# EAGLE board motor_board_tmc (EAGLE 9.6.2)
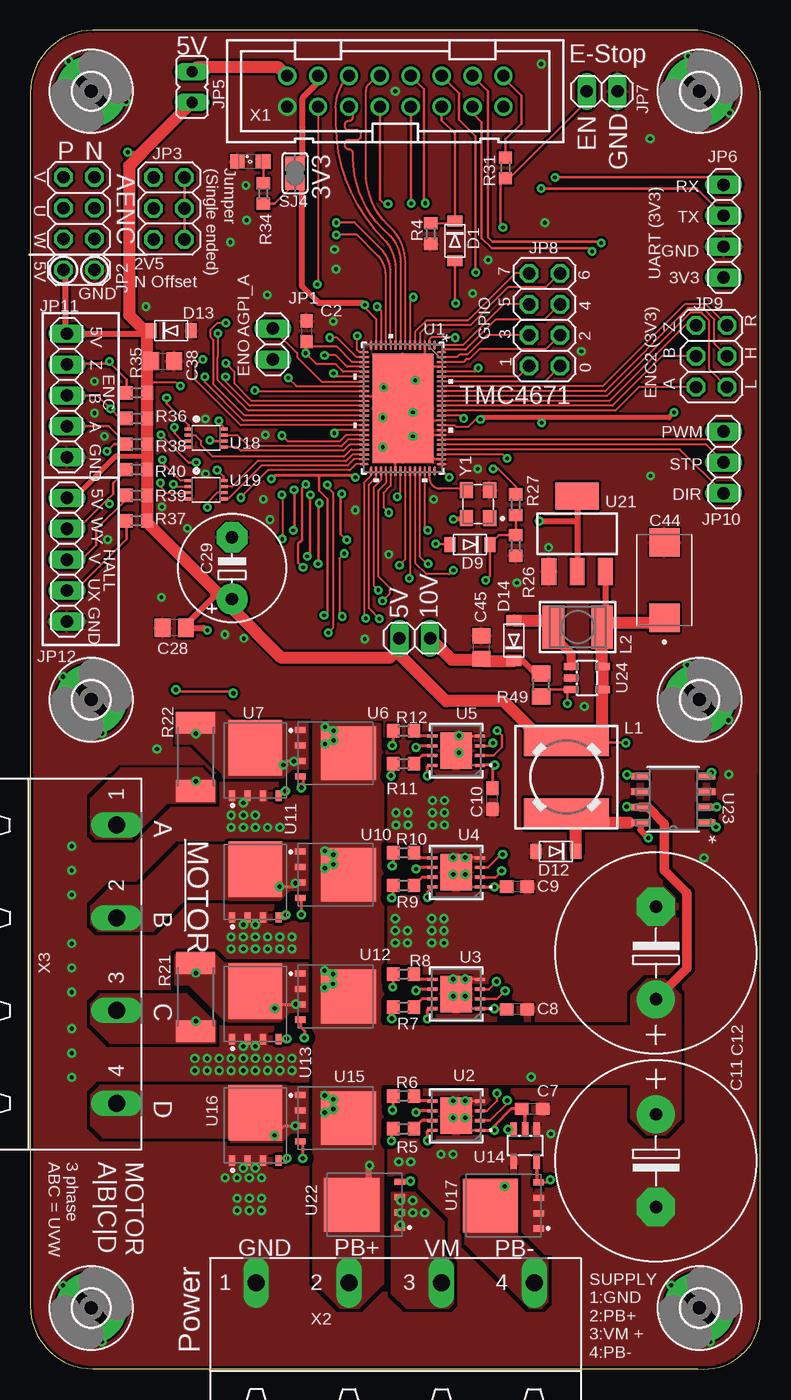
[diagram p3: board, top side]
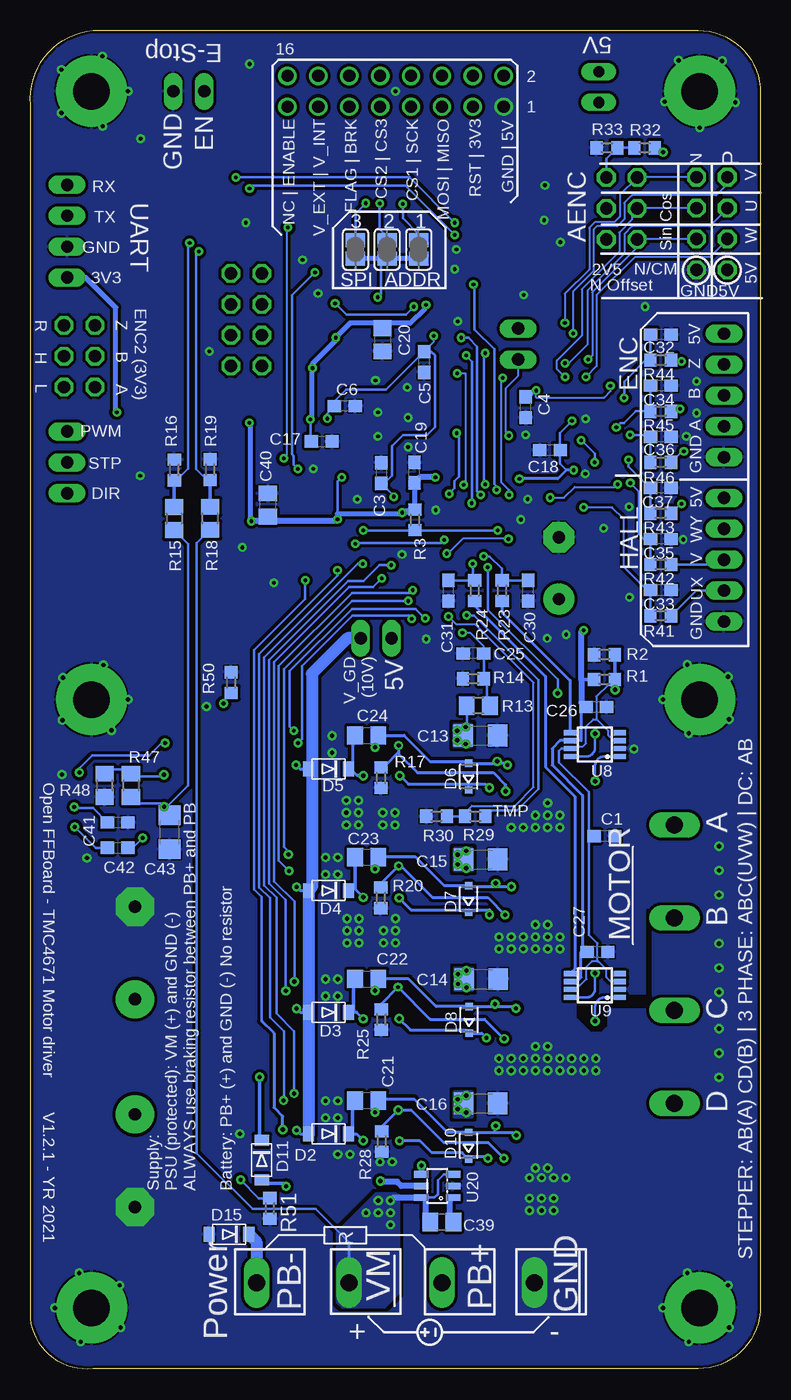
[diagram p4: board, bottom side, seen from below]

Size 60.02 x 110.03 mm. Coordinates in mm from the lower left corner, seen from the top.
Outline: 0,104.91 0,5.15 arc90 5.12,0.03 54.88,0.03 arc90 60,4.15 60,103.91 arc90 54.88,110.03 5.12,110.03 arc90 0,104.91
Copper layers (1*16): Top 0.035mm / dielectric 1.5mm / Bottom 0.035mm
Design rules "jlcpcb *": minimum track width 5mil, minimum drill 0.3mm, track to track 8mil, track to pad 8mil, pad to pad 8mil, via to via 8mil, smd to smd 5mil, copper to edge 0.2mm, drill to drill 8mil, minimum pad ring 10mil, minimum via ring 8mil, stop-mask expansion 4mil, vias tented up to drill 0.4mm, thermal gap 6mil

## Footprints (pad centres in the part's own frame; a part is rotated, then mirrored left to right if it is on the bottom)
C0603 = smd 1.1 x 1: 1 -0.85,0; 2 0.85,0
E7,5-16 = drill 1.016 pad 3.15: + -3.81,0 | drill 1.016 pad 3.15 octagon: - 3.81,0
C1206 = smd 1.6 x 1.8: 1 -1.4,0; 2 1.4,0
C0805 = smd 1.3 x 1.5: 1 -0.95,0; 2 0.95,0
E5-8,5 = drill 1.016 pad 2.54: + -2.54,0 | drill 1.016 pad 2.54 octagon: - 2.54,0
CAPPM7343X310N = smd 2.31 x 2.52: 1 -3.1,0; 2 3.1,0
SOD-123FL = smd 0.91 x 1.22: A 1.637,0; C -1.637,0
SOD323-R = smd 0.6 x 0.6: A 1.1,0; C -1.1,0
3,0-PAD = drill 3 pad 5.842: B3,0 0,0
1X02 = drill 1.016 long: 1 -1.27,0; 2 1.27,0
2X04 = drill 1.016 octagon: 1 -3.81,-1.27; 2 -3.81,1.27; 3 -1.27,-1.27; 4 -1.27,1.27; 5 1.27,-1.27; 6 1.27,1.27; 7 3.81,-1.27; 8 3.81,1.27
2X03 = drill 1.016 octagon: 1 -2.54,-1.27; 2 -2.54,1.27; 3 0,-1.27; 4 0,1.27; 5 2.54,-1.27; 6 2.54,1.27
JP1 = drill 0.914 long: 1 0,-1.27; 2 0,1.27
1X04 = drill 1.016 long: 1 -3.81,0; 2 -1.27,0; 3 1.27,0; 4 3.81,0
1X03 = drill 1.016 long: 1 -2.54,0; 2 0,0; 3 2.54,0
1X05 = drill 1.016 long: 1 -5.08,0; 2 -2.54,0; 3 0,0; 4 2.54,0; 5 5.08,0
8MMINDUCTOR = smd 2.5 x 7: 1 -3,0; 2 3,0
L4532P = smd 1.8 x 3.6: 1 -2,0; 2 2,0
SML0805 = smd 1.2 x 1.2: A 1.05,0; C -1.05,0
R0603 = smd 1 x 1.1: 1 -0.85,0; 2 0.85,0
R0805 = smd 1.3 x 1.5: 1 -0.95,0; 2 0.95,0
R2512 = smd 1.8 x 3.2: 1 -2.8,0; 2 2.8,0
SJ = smd 1.168 x 1.6: 1 -0.762,0; 2 0.762,0
QFN76_10P5X6P5 = smd 0.152 x 0.755: 1 -2.6,-5.173; 2 -2.2,-5.173; 3 -1.8,-5.173; 4 -1.4,-5.173; 5 -1,-5.173; 6 -0.6,-5.173; 7 -0.2,-5.173; 8 0.2,-5.173; 9 0.6,-5.173; 10 1,-5.173; 11 1.4,-5.173; 12 1.8,-5.173; 13 2.2,-5.173; 14 2.6,-5.173; 39 2.6,5.173; 40 2.2,5.173; 41 1.8,5.173; 42 1.4,5.173; 43 1,5.173; 44 0.6,5.173; 45 0.2,5.173; 46 -0.2,5.173; 47 -0.6,5.173; 48 -1,5.173; 49 -1.4,5.173; 50 -1.8,5.173; 51 -2.2,5.173; 52 -2.6,5.173 | smd 0.755 x 0.152: 15 3.179,-4.6; 16 3.179,-4.2; 17 3.179,-3.8; 18 3.179,-3.4; 19 3.179,-3; 20 3.179,-2.6; 21 3.179,-2.2; 22 3.179,-1.8; 23 3.179,-1.4; 24 3.179,-1; 25 3.179,-0.6; 26 3.179,-0.2; 27 3.179,0.2; 28 3.179,0.6; 29 3.179,1; 30 3.179,1.4; 31 3.179,1.8; 32 3.179,2.2; 33 3.179,2.6; 34 3.179,3; 35 3.179,3.4; 36 3.179,3.8; 37 3.179,4.2; 38 3.179,4.6; 53 -3.179,4.6; 54 -3.179,4.2; 55 -3.179,3.8; 56 -3.179,3.4; 57 -3.179,3; 58 -3.179,2.6; 59 -3.179,2.2; 60 -3.179,1.8; 61 -3.179,1.4; 62 -3.179,1; 63 -3.179,0.6; 64 -3.179,0.2; 65 -3.179,-0.2; 66 -3.179,-0.6; 67 -3.179,-1; 68 -3.179,-1.4; 69 -3.179,-1.8; 70 -3.179,-2.2; 71 -3.179,-2.6; 72 -3.179,-3; 73 -3.179,-3.4; 74 -3.179,-3.8; 75 -3.179,-4.2; 76 -3.179,-4.6 | smd 5.004 x 8.992: 77 0,0
SDC08A = smd 0.254 x 0.813: 1 -1.2,-1.943; 2 -0.4,-1.943; 3 0.4,-1.943; 4 1.2,-1.943; 5 1.2,1.943; 6 0.4,1.943; 7 -0.4,1.943; 8 -1.2,1.943 | smd 2.997 x 2.591: 9 0,0
MOSFET_BSC093N04LSGATMA1 = smd 0.5 x 0.85: 1 -1.905,-2.9; 2 -0.635,-2.9; 3 0.635,-2.9; 4 1.905,-2.9 | smd 4.41 x 4.55: 5 0,1.05
MSOP8 = smd 0.432 x 0.991: 1 -0.975,-2.05; 2 -0.325,-2.05; 3 0.325,-2.05; 4 0.975,-2.05; 5 0.975,2.05; 6 0.325,2.05; 7 -0.325,2.05; 8 -0.975,2.05
SOT23-5L = smd 0.55 x 1.2: 1 -0.95,-1.3; 2 0,-1.3; 3 0.95,-1.3; 4 0.95,1.3; 5 -0.95,1.3
VFSOP-8 = smd 0.25 x 0.65: P$1 -0.75,-1.45; P$2 -0.25,-1.45; P$3 0.25,-1.45; P$4 0.75,-1.45; P$5 0.75,1.45; P$6 0.25,1.45; P$7 -0.25,1.45; P$8 -0.75,1.45
SOT23-6 = smd 0.55 x 1.2: 1 -0.95,-1.3; 2 0,-1.3; 3 0.95,-1.3; 4 0.95,1.3; 5 0,1.3; 6 -0.95,1.3
SOT223 = smd 1.219 x 2.235: 1 -2.311,-3.099; 2 0,-3.099; 3 2.311,-3.099 | smd 3.6 x 2.2: 4 0,3.099
21-0041B_8_MXM = smd 0.543 x 1.455: 1 -1.905,-2.721; 2 -0.635,-2.721; 3 0.635,-2.721; 4 1.905,-2.721; 5 1.905,2.721; 6 0.635,2.721; 7 -0.635,2.721; 8 -1.905,2.721
PAK100/2500-16 = drill 1 pad 1.422: 1 -8.89,-1.27; 2 -8.89,1.27; 3 -6.35,-1.27; 4 -6.35,1.27; 5 -3.81,-1.27; 6 -3.81,1.27; 7 -1.27,-1.27; 8 -1.27,1.27; 9 1.27,-1.27; 10 1.27,1.27; 11 3.81,-1.27; 12 3.81,1.27; 13 6.35,-1.27; 14 6.35,1.27; 15 8.89,-1.27; 16 8.89,1.27
GMSTBA4 = drill 1.397 long: 1 -11.43,5.08; 2 -3.81,5.08; 3 3.81,5.08; 4 11.43,5.08
ECS-327KE-TR = smd 1.3 x 1.1: 1 -1.15,-0.95; 2 1.15,-0.95; 3 1.15,0.95; 4 -1.15,0.95

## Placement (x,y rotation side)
C1  100nF  [C0603]  12.82,43.8 180 bottom
C2  100nF  [C0603]  22.7,85.3 270 top
C3  100nF  [C0603]  31.18,73.65 270 bottom
C4  100nF  [C0603]  19.3,79.05 90 bottom
C5  100nF  [C0603]  27.65,82.78 90 bottom
C6  100nF  [C0603]  34.17,79.15 180 bottom
C7  100nF  [C0603]  41.25,21.38 180 top
C8  100nF  [C0603]  40,29.58 180 top
C9  100nF  [C0603]  40,39.65 180 top
C10  100nF  [C0603]  37.98,46.88 90 top
C11  680µF  [E7,5-16]  51.42,17.13 270 top
C12  680µF  [E7,5-16]  51.42,34.2 90 top
C13  1µF  [C1206]  23.02,52.08 0 bottom
C14  1µF  [C1206]  22.98,32.05 0 bottom
C15  1µF  [C1206]  23,41.88 0 bottom
C16  1µF  [C1206]  23,21.83 0 bottom
C17  100nF  [C0603]  36.08,76.25 0 bottom
C18  100nF  [C0603]  17.3,75.53 180 bottom
C19  100nF  [C0603]  28.45,73.68 90 bottom
C20  4.7µF  [C0805]  31.07,84.6 270 bottom
C21  100nF  [C0805]  32.38,22.08 0 bottom
C22  100nF  [C0805]  32.38,32.08 0 bottom
C23  100nF  [C0805]  32.38,42.08 0 bottom
C24  100nF  [C0805]  32.38,52.08 0 bottom
C25  1n  [C0603]  23.6,58.83 180 bottom
C26  100nF  [C0603]  13.5,54.43 0 bottom
C27  100nF  [C0603]  13.4,34.3 0 bottom
C28  4.7µF  [C0805]  11.82,60.93 180 top
C29  [E5-8,5]  16.57,65.83 90 top
C30  1n  [C0603]  19.1,63.98 90 bottom
C31  1n  [C0603]  25.65,63.98 90 bottom
C32  100p  [C0603]  8.2,85.03 180 bottom
C33  1n  [C0603]  8.2,64.03 180 bottom
C34  100p  [C0603]  8.2,80.83 180 bottom
C35  1n  [C0603]  8.2,68.23 180 bottom
C36  100p  [C0603]  8.2,76.63 180 bottom
C37  1n  [C0603]  8.2,72.43 180 bottom
C38  4.7µF  [C0805]  10.88,82.85 0 top
C39  100nF  [C0805]  26.2,12.08 180 bottom
C40  4.7µF  [C0805]  40.5,71.03 90 bottom
C41  100nF  [C0603]  52.85,44.93 180 bottom
C42  100nF  [C0603]  52.85,42.85 0 bottom
C43  1µF  [C1206]  48.58,44.13 90 bottom
C44  593D476X0016D2TE3  [CAPPM7343X310N]  52.12,64.85 90 top
C45  4.7µF <REMOVE>  [C0805]  37.08,59.33 90 top
D1  LV low drop  [SOD-123FL]  34.9,92.73 270 top
D2  HV >100V  [SOD-123FL]  35.5,19.33 180 bottom
D3  HV >100V  [SOD-123FL]  35.5,29.33 180 bottom
D4  HV >100V  [SOD-123FL]  35.5,39.33 180 bottom
D5  HV >100V  [SOD-123FL]  35.5,49.33 180 bottom
D6  BZX384-XXX  [SOD323-R]  24,48.7 90 bottom
D7  BZX384-XXX  [SOD323-R]  24,38.63 90 bottom
D8  BZX384-XXX  [SOD323-R]  23.95,28.7 90 bottom
D9  LV low drop  [SOD-123FL]  36.12,67.78 180 top
D10  BZX384-XXX  [SOD323-R]  24,18.35 90 bottom
D11  HV >100V  [SOD-123FL]  41,17.18 270 bottom
D12  HV >100V  [SOD-123FL]  43.2,42.55 180 top
D13  5.6V zener  [SOD-123FL]  11.57,85.35 0 top
D14  LV low drop  [SOD-123FL]  39.75,59.88 90 top
D15  Zener 65V (MMSZ5265BT1G)  [SOD-123FL]  43.7,11.08 180 bottom
H1  MOUNT-PAD-ROUND3.0  [3,0-PAD]  55,5.03 0 top
H2  MOUNT-PAD-ROUND3.0  [3,0-PAD]  5,5.03 0 top
H3  MOUNT-PAD-ROUND3.0  [3,0-PAD]  55,105.03 0 top
H4  MOUNT-PAD-ROUND3.0  [3,0-PAD]  55,55.03 0 top
H5  MOUNT-PAD-ROUND3.0  [3,0-PAD]  5,105.03 0 top
H6  MOUNT-PAD-ROUND3.0  [3,0-PAD]  5,55.03 0 top
JP1  [1X02]  19.93,84.25 90 top
JP2  [2X04]  4,94.15 90 top
JP3  [2X03]  11.4,95.4 270 top
JP4  V_DRV  [1X02]  31.6,60.08 180 top
JP5  5V  [JP1]  13.3,105.38 180 top
JP6  [1X04]  57,93.53 270 top
JP7  [1X02]  47,105.03 180 top
JP8  [2X04]  42.27,86.25 90 top
JP9  [2X03]  56,83.25 90 top
JP10  [1X03]  57,74.53 270 top
JP11  [1X05]  3,80.03 270 top
JP12  [1X05]  3,66.53 270 top
L1  220µH  [8MMINDUCTOR]  44.08,48.65 90 top
L2  10µH  [L4532P]  45,60.98 180 top
LED1  Green  [SML0805]  18.07,99.25 0 top
R1  10k  [R0603]  12.82,56.68 180 bottom
R2  10k  [R0603]  12.82,58.73 0 bottom
R3  10k  [R0603]  28.4,69.8 90 bottom
R4  10k  [R0603]  32.9,93.33 90 top
R5  2.2  [R0603]  30.68,19.75 0 top
R6  2.2  [R0603]  30.68,22.45 0 top
R7  2.2  [R0603]  30.68,29.75 0 top
R8  2.2  [R0603]  30.68,32.45 0 top
R9  2.2  [R0603]  30.68,39.75 0 top
R10  2.2  [R0603]  30.68,42.45 0 top
R11  2.2  [R0603]  30.68,49.75 0 top
R12  2.2  [R0603]  30.68,52.45 0 top
R13  71.5k  [R0805]  23.2,54.53 180 bottom
R14  1.5k  [R0603]  23.6,56.75 0 bottom
R15  294k  [R0805]  48.2,69.9 270 bottom
R16  10k  [R0603]  48.2,73.9 270 bottom
R17  33k  [R0603]  31.2,48.6 90 bottom
R18  294k  [R0805]  45.25,69.93 270 bottom
R19  10k  [R0603]  45.25,73.93 270 bottom
R20  33k  [R0603]  31.23,38.73 90 bottom
R21  1.5m  [R2512]  13.6,30.58 90 top
R22  1.5m  [R2512]  13.6,50.33 90 top
R23  1.5k  [R0603]  21.25,63.98 270 bottom
R24  1.5k  [R0603]  23.5,63.98 270 bottom
R25  33k  [R0603]  31.18,28.73 90 bottom
R26  10k  [R0603]  39.9,67.7 90 top
R27  1.5k  [R0603]  39.9,71.05 270 top
R28  33k  [R0603]  31.15,18.7 90 bottom
R29  22k thermistor  [R0603]  23.45,45.43 0 bottom
R30  1.5k  [R0603]  26.62,45.43 0 bottom
R31  1.5k  [R0603]  39.05,98.73 90 top
R32  10k  [R0603]  9.53,100.38 0 bottom
R33  10k  [R0603]  12.62,100.38 0 bottom
R34  330  [R0603]  19.15,96.63 270 top
R35  4.7k  [R0603]  8.75,80.23 0 top
R36  4.7k  [R0603]  8.75,78.13 0 top
R37  4.7k  [R0603]  8.75,69.73 0 top
R38  4.7k  [R0603]  8.75,76.03 0 top
R39  4.7k  [R0603]  8.75,71.83 0 top
R40  4.7k  [R0603]  8.75,73.93 0 top
R41  1.5k  [R0603]  8.2,61.93 0 bottom
R42  1.5k  [R0603]  8.2,66.13 0 bottom
R43  1.5k  [R0603]  8.2,70.33 0 bottom
R44  1.5k  [R0603]  8.2,82.93 0 bottom
R45  1.5k  [R0603]  8.2,78.73 0 bottom
R46  1.5k  [R0603]  8.2,74.53 0 bottom
R47  294k  [R0805]  51.75,47.98 270 bottom
R48  71.5k  [R0805]  53.92,47.98 270 bottom
R49  71.5k  [R0805]  42,56.23 90 top
R50  10k  [R0603]  43.52,56.43 270 bottom
R51  33k  [R0603]  40.33,13.2 90 bottom
SJ1  [SJ]  28.1,92.03 270 bottom
SJ2  [SJ]  30.7,92.03 270 bottom
SJ3  [SJ]  33.3,92.03 270 bottom
SJ4  3.3V  [SJ]  21.75,98.3 270 top
U1  TMC4671  [QFN76_10P5X6P5]  30.62,78.98 180 top
U2  LM5109BSD  [SDC08A]  35,20.83 90 top
U3  LM5109BSD  [SDC08A]  35,30.83 90 top
U4  LM5109BSD  [SDC08A]  35,40.83 90 top
U5  LM5109BSD  [SDC08A]  35,50.83 90 top
U6  BSC030N08NS5ATMA1  [MOSFET_BSC093N04LSGATMA1]  25.1,50.63 270 top
U7  BSC030N08NS5ATMA1  [MOSFET_BSC093N04LSGATMA1]  18.5,50.03 0 top
U8  AD841X  [MSOP8]  13.6,51.33 90 bottom
U9  AD841X  [MSOP8]  13.6,31.53 90 bottom
U10  BSC030N08NS5ATMA1  [MOSFET_BSC093N04LSGATMA1]  25.1,40.63 270 top
U11  BSC030N08NS5ATMA1  [MOSFET_BSC093N04LSGATMA1]  18.5,40.03 0 top
U12  BSC030N08NS5ATMA1  [MOSFET_BSC093N04LSGATMA1]  25.1,30.63 270 top
U13  BSC030N08NS5ATMA1  [MOSFET_BSC093N04LSGATMA1]  18.5,30.03 0 top
U14  MCP14XX  [SOT23-5L]  40.67,18.38 180 top
U15  BSC030N08NS5ATMA1  [MOSFET_BSC093N04LSGATMA1]  25.1,20.63 270 top
U16  BSC030N08NS5ATMA1  [MOSFET_BSC093N04LSGATMA1]  18.5,20.03 0 top
U17  BSC030N08NS5ATMA1  [MOSFET_BSC093N04LSGATMA1]  38.88,13.45 90 top
U18  NC7NZ17K8X-3-BUFFER  [VFSOP-8]  14.45,76.53 270 top
U19  NC7NZ17K8X-3-BUFFER  [VFSOP-8]  14.45,72.28 270 top
U20  LM74700-Q1  [SOT23-6]  26.57,15.05 90 bottom
U21  [SOT223]  44.95,68.65 0 top
U22  BSC030N08NS5ATMA1  [MOSFET_BSC093N04LSGATMA1]  27.48,13.5 90 top
U23  MAX5033BASA+T  [21-0041B_8_MXM]  52.85,46.83 90 top
U24  AP3012KTR-G1  [SOT23-5L]  45.75,56.8 270 top
X1  2516-  [PAK100/2500-16]  30,105.03 0 top
X2  GMSTBA4  [GMSTBA4]  30,2.03 0 top
X3  GMSTBA4  [GMSTBA4]  2,33.28 270 top
Y1  25MHz  [ECS-327KE-TR]  36.8,71.1 90 top

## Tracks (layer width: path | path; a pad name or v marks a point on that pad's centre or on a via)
+3V3  (via drill 0.3)
  Top 0.152: U1.52 33.25,73.78 33.95,73.78 v34.42,73.3 | U1.43 29.62,72.6 29.02,72 29.02,70.83 v29.45,70.4 | U1.13 28.42,86.3 27.5,87.22 v27.5,87.48 | v34.92,84.78 34.92,84.83 33,84.83 32.82,84.65 U1.2 | v36.83,82.28 36.52,81.98 U1.72 | v37,78.05 36.6,78.05 35.99,77.44 35,77.44 34.87,77.58 U1.61
  Top 0.2: U18.P$8 15.96,77.34 15.5,77.8 v15.5,77.93 | v15.35,73.89 15.9,73.34 U19.P$8 | R34.2 20.07,95.78 21.75,97.45 SJ4.2 | v24.14,61.95 24.43,62.24 24.43,71.49 23.73,72.2 23.73,73.45
  Top 0.254: v26.73,73.3 26.57,73.45 23.73,73.45 20.09,73.45 v19.82,73.18
  Top 0.4: Y1.4 35.75,69.85 v34.77,69.85 | v52.92,78.63 52.5,78.2 42.05,78.2 | 42.05,78.2 37.15,78.2 v37,78.05 | v42.02,77.78 42.02,78.18 42.05,78.2
  Top 0.5: v27.5,87.48 27.32,87.65 23.68,87.65 22.3,89.03 22.3,96.99 SJ4.2 | U21.4 44.95,69.7 | v41.85,69.7 44.95,69.7 | 44.95,69.7 U21.2
  Bottom 0.152: C18.1 16.45,75.58 16.5,75.63
  Bottom 0.2: v15.35,73.89 15.97,73.89 16.5,74.42 16.5,75.63 16.5,76.93 v15.5,77.93 | R3.2 29.2,70.65 v29.45,70.4 | C40.1 40.88,69.7 v41.85,69.7 | v34.42,73.3 34.77,72.95 v34.77,69.85 | C17.1 37,76.33 v37,78.05 | R29.2 22.1,45.92 20.02,45.92 18.27,47.67 18.27,56.65 23.57,61.95 v24.14,61.95
  Bottom 0.254: v15.35,73.89 15.95,73.89 16.66,73.18 v19.82,73.18
  Bottom 0.3: v27.5,87.48 27.6,87.38 | v36.83,82.28 36.91,82.2 | v37,78.05 36.91,78.15 | v34.77,69.85 34.77,69.73 | 34.92,84.53 v34.92,84.78
  Bottom 0.4: v34.77,69.85 34.77,70.3 29.55,70.3 v29.45,70.4 29.07,70.4 28.45,71.03 C19.1 | 27.6,87.38 27.6,87.13 28.77,85.95 31.07,85.95 | 36.91,82.2 36.91,78.15 | v52.92,78.63 53,78.7 53,87.25 55.47,89.72 JP6.4 | v34.92,84.78 33.73,85.98 31.07,85.98 31.07,85.95 | v42.02,77.78 41.98,77.73 41.98,69.83 v41.85,69.7 | C20.1 31.07,85.95 | v36.83,82.28 36.83,82.63 34.92,84.53
  Bottom 0.5: v41.85,69.7 41.83,69.73 34.77,69.73 | v26.73,73.3 27.98,73.3 C19.1
+5V  (via drill 0.3, 0.35)
  Top 0.152: U1.23 18.5,80.38 v18.45,80.43 | R35.2 9.6,80.88 9.82,81.1 11.93,81.1 12.21,80.81 v12.34,80.81
  Top 0.2: D13.C 9.6,85.35 9.6,85.13 | U23.4 55.9,48.73 56,48.84 v56,49.03 | v48.95,51.45 48.91,51.49 47.54,51.49 47.38,51.65 L1.2 | v8,100.03 9,100.03 9.11,99.92
  Top 0.4: JP12.1 3.58,71.61 7.03,75.05 9.6,75.05
  Top 0.5: 9.6,85.13 9.58,85.11 JP11.1 2.88,85.23 2.88,90.2 JP2.2 | U24.4 47,55.8 | 47,52.03 46.62,51.65 L1.2 | v14.55,60.73 14.4,60.73 14.2,60.93 C28.1 12.78,61.14 15.07,63.44 15.07,64.1 | C29.+ 16.55,63.26 16.55,62.63
  Top 0.508: U21.3 47.26,61.24 L2.1
  Top 0.8: U24.5 47,57.8
  Top 1: U24.4 U24.5 | 9.6,83.03 R35.2 R36.2 R38.2 9.6,75.05 R40.2 R39.2 R37.2 9.6,69.58 15.07,64.1 16.55,62.63 | 9.6,83.03 9.6,85.13 8.1,86.63 8.1,98.91 9.11,99.92 JP5.2 | 47,55.8 47,52.03 | L1.2 42.12,51.65 38.88,54.9 34.18,54.9 30.33,58.75 JP4.2 30.33,59.25 29.54,58.46 20.66,58.46 16.55,62.58 16.55,63.26 | C38.1 9.75,83.03 9.6,83.03 | C44.1 51.67,61.3 47.33,61.3 L2.1 47,57.8
  Bottom 0.152: C4.2 18.98,79.9 v18.45,80.43 18.45,79.86 12.84,79.86 12.34,80.36 v12.34,80.81
  Bottom 0.2: v56,49.03 56,49.38 54.95,50.43 50.27,50.43 49.25,51.45 v48.95,51.45 | R32.2 8.32,100.03 v8,100.03
  Bottom 0.25: U8.6 16.48,51.65
  Bottom 0.254: C26.1 14.75,54.03 14.75,51.65 U8.6 | 16.48,51.65 17.12,51 17.12,49.65 14.62,47.15 14.62,34.68 C27.1 14.75,34.3 14.75,32.2 15.1,31.85 U9.6
  Bottom 0.3: R1.2 14.7,56.68 14.72,56.65
  Bottom 0.5: C26.1 14.72,54.8 14.72,56.65 14.72,60.55 v14.55,60.73
AENC_UX  (via drill 0.3)
  Top 0.15: 18.2,79.58 16.75,81.03 16.75,82 v16.07,82.68
  Top 0.152: U1.25 18.2,79.58
  Bottom 0.15: 14.22,88.65 14.22,84.2 15.75,82.68 v16.07,82.68
  Bottom 0.152: 14.22,88.65 11.19,91.69 11.19,93.29 10.56,93.93 4.17,93.93 2.73,95.37 JP2.6
AENC_UX_N  (via drill 0.3)
  Top 0.15: U1.26 18.02,79.18 16.05,81.15 v16.05,81.55
  Bottom 0.152: v16.05,81.55 16.1,81.55 16.75,82.2 16.75,82.9 14.7,84.95 14.7,88.75 11.61,91.84 11.61,93.42 10.58,94.45 10.58,94.95 JP3.3 10.11,95.42 JP2.5
AENC_VN  (via drill 0.3)
  Top 0.15: U1.27 17.91,78.78
  Top 0.152: 17.91,78.78 15.39,81.29 15.39,83.17 15.41,83.18 v15.41,85.13
  Bottom 0.152: 2.72,97.41 3.65,96.48 10.57,96.48 11.2,95.85 11.2,94.5 11.78,93.92 13.46,93.92 13.72,93.65 13.72,90.23 15.41,88.55 v15.41,85.13
  Bottom 0.2: JP2.8 2.72,97.95 2.72,97.41
AENC_VN_N  (via drill 0.3)
  Top 0.15: U1.28 17.62,78.38 15.04,80.96
  Top 0.152: v16.08,85.98 15.36,85.98 14.78,85.4 14.78,84.87 15.04,84.61 15.04,80.96
  Bottom 0.152: v16.08,85.98 16.08,88.38 14.08,90.38 14.08,93.8 13.61,94.27 12.01,94.27 11.56,94.72 11.56,96.52 JP3.1 10.11,97.96 JP2.7
AENC_WY  (via drill 0.3)
  Top 0.15: U1.29 17.48,77.98 14.35,81.11 v14.35,81.55
  Bottom 0.152: v14.35,81.55 13.47,82.43 13.47,88.25 10.32,91.4 4.16,91.4 2.73,92.83 JP2.4
AENC_WY_N  (via drill 0.3)
  Top 0.15: U1.30 17.28,77.58 13.57,81.28 13.57,82.53
  Top 0.152: 13.57,82.53 14.03,82.98 v14.17,82.98
  Bottom 0.152: v14.17,82.98 13.83,83.31 13.83,88.5 10.13,92.2 JP3.5 10.11,92.88 JP2.3
AGPI_A
  Top 0.152: U1.21 23.93,81.18 21.93,83.18 21.93,83.52 JP1.2
AGPI_B  (via drill 0.3)
  Top 0.152: v21.19,81.47 v21.19,81.46 21.88,80.78 U1.22 | v20.68,71.85 20.73,71.8 v20.73,68.23 | v25.65,61.85 25.41,62.09 25.41,66.64 v25.8,67.03
  Bottom 0.152: v21.19,81.47 21.19,81.34 21.32,81.22 21.32,72.9 20.68,72.25 v20.68,71.85 | v20.73,68.23 20.75,68.25 24.48,68.25 25.7,67.03 v25.8,67.03 | R29.1 24.3,45.73 23.73,46.3 20.18,46.3 18.65,47.83 18.65,56.42 23.44,61.21 25.01,61.21 v25.65,61.85
  Bottom 0.2: R29.1 R30.2
BRAKE_CTRL  (via drill 0.3, 0.35)
  Top 0.2: R27.2 R26.2 38.54,68.55 D9.C 37.76,65.16 v37.42,64.83
  Top 0.254: U14.3 v39.27,19.68
  Bottom 0.2: 41,28.63 41,38.82 41.62,39.43 41.62,59.09 37.42,63.28 v37.42,64.83
  Bottom 0.254: v39.27,19.68 39.27,20.78 40,21.5 40,27.63 41,28.63
BRAKE_CTRL_EXT  (via drill 0.3)
  Top 0.2: X1.12 35.25,104.86 35.25,102.68 36.6,101.33 36.6,90.18 v36.62,90.15 | R27.1 39.9,72.54 38.44,74 v38.03,74
  Bottom 0.2: v38.03,74 38.38,74.35 38.38,75.05 38.52,75.19 38.52,88.26 v36.62,90.15
BRAKE_CTRL_TMC  (via drill 0.3)
  Top 0.152: U1.31 25.23,77.18 v24.98,76.93
  Top 0.2: D9.A 34.44,67.83 v33.33,67.83 | v25.6,71.95 25.5,71.85 25.5,68.65 v26,68.15
  Bottom 0.2: v24.98,76.93 24.8,76.75 24.8,73.35 25.15,73 25.15,72.4 v25.6,71.95 | v33.33,67.83 33.25,67.9 26.25,67.9 v26,68.15
BRAKE_GATE  (via drill 0.35)
  Top 0.2: v42.75,15.55 42.55,15.36 U17.4
  Top 0.3: U17.4 41.65,15.48 41.65,17.05 U14.5
  Bottom 0.2: R51.2 41.25,14.05 v42.75,15.55
C_HS_A  (via drill 0.3)
  Top 0.152: U1.39 28.02,73.45 27.42,72.85 27.42,61.85 v27.57,61.7
  Top 0.2: U5.2 38.08,50.43 38.77,51.13 38.77,52.08 v38.38,52.48
  Bottom 0.2: v38.38,52.48 38.7,52.8 38.7,57.37 33.59,62.48 28.34,62.48 v27.57,61.7
C_HS_B  (via drill 0.3, 0.35)
  Top 0.152: U1.41 28.82,73.05 28.22,72.45 28.22,64.41 v28.6,64.03
  Top 0.2: U4.2 38.23,40.43 v38.75,40.95
  Bottom 0.2: v38.75,40.95 39.6,41.8 39.6,57.8 33.6,63.8 28.82,63.8 v28.6,64.03
C_HS_C  (via drill 0.3, 0.35)
  Top 0.152: U1.46 30.8,73.78 30.8,66.53 v30.34,66.08
  Top 0.2: U3.2 38.38,30.43 v39.02,31.08
  Bottom 0.2: v39.02,31.08 39.02,38.55 40.41,39.93 40.41,58.27 33.91,64.76 32.64,64.76 31.32,66.08 v30.34,66.08
C_HS_D  (via drill 0.3, 0.35)
  Top 0.152: v34.77,65.65 34.45,65.33 32.55,65.33 31.62,66.26 U1.48
  Top 0.2: U2.2 37.77,20.43 39.2,21.85 v39.2,22.08
  Bottom 0.2: v39.2,22.08 39.15,22.13 39.15,27.75 40.33,28.93 40.33,38.71 41.21,39.6 41.21,58.79 34.77,65.23 v34.77,65.65
C_LS_A  (via drill 0.3, 0.35)
  Top 0.152: U1.40 28.42,73.3 27.82,72.7 27.82,62.53 v28.68,61.68
  Top 0.2: U5.3 37.8,51.23 v38.02,51.45
  Bottom 0.2: v38.02,51.45 37.7,51.78 37.7,57.78 33.52,61.95 28.68,61.95 v28.68,61.68
C_LS_B  (via drill 0.3, 0.35)
  Top 0.152: U1.42 29.22,72.8 28.62,72.2 28.62,65.13 29.56,64.19 29.56,63.74 v28.95,63.13
  Top 0.2: U4.3 37.62,41.23 38.7,42.3 v38.83,42.3
  Bottom 0.2: v38.83,42.3 38.83,42.58 39.15,42.9 39.15,57.55 33.57,63.13 v28.95,63.13
C_LS_C  (via drill 0.3, 0.35)
  Top 0.152: U1.47 31.22,65.05 v31.15,64.98
  Top 0.2: U3.3 37.7,31.23 v38.33,31.85
  Bottom 0.2: v38.33,31.85 38.33,38.42 40,40.1 40,58.1 33.82,64.28 31.85,64.28 v31.15,64.98
C_LS_D  (via drill 0.3, 0.35)
  Top 0.152: U1.49 32,73.78 32,66.78 32.58,66.2 v32.7,66.2
  Top 0.2: v38.35,22.65 38.35,22.05 37.52,21.23 U2.3
  Bottom 0.2: v38.35,22.65 38.35,27.78 39.8,29.23 39.8,38.76 40.81,39.77 40.81,58.49 33.1,66.2 v32.7,66.2
CLK_25M
  Top 0.152: Y1.3 35.75,72.35 33.7,72.35 arc-90 32.82,73.23 U1.51
CS1  (via drill 0.3)
  Top 0.2: X1.7 28.73,96.12 29.1,95.75 v29.4,95.75
  Bottom 0.2: SJ1.1 28.1,93.29 29.4,94.59 v29.4,95.75
CS2  (via drill 0.3)
  Top 0.2: X1.9 31.27,95.84 v31.3,95.81
  Bottom 0.2: v31.3,95.81 31.3,93.71 30.7,93.11 SJ2.1
CS3  (via drill 0.3)
  Top 0.2: X1.10 32.38,105.19 32.38,95.8 32.42,95.8 v32.45,95.83
  Bottom 0.2: SJ3.1 33.3,94.98 v32.45,95.83
CS_TMC  (via drill 0.3)
  Top 0.152: 31.43,88.1 31.22,87.9 U1.6
  Top 0.2: v31.48,88.1 31.43,88.1
  Bottom 0.2: v31.48,88.1 31.2,88.38 31.2,90.76 SJ2.2
  Bottom 0.4: SJ1.2 SJ2.2 SJ3.2
DIR
  Top 0.152: JP10.3 53.41,75.58 U1.56
ENABLE  (via drill 0.3)
  Top 0.152: U1.55 38.87,75.18 v39.2,74.84
  Top 0.2: v38.85,93.82 38.62,94.05 38.62,97.45 R31.1 39.4,97.88 45.73,104.21 JP7.2
  Bottom 0.152: v38.85,93.82 38.95,93.72 38.95,75.09 v39.2,74.84
ENC2_A
  Top 0.152: JP9.2 50.03,80.71 48.09,78.78 U1.64
ENC2_B
  Top 0.152: JP9.4 51.93,83.25 47.85,79.18 U1.65
ENC2_Z
  Top 0.152: JP9.6 53.83,85.79 47.62,79.58 U1.66
ENC_A
  Top 0.152: U1.35 26.37,75.58 25.78,74.99 14.99,74.99 14.04,75.94 14.04,76.29 13.6,76.73 13.05,76.73 U18.P$2
ENC_A_5V  (via drill 0.3)
  Top 0.2: U18.P$6 14.8,76.28 v14.75,76.33 | v13.62,74.53 13,74.53 10.75,76.78 v10.72,76.78
  Bottom 0.152: C36.2 9.2,76.78
  Bottom 0.2: v14.75,76.33 14.7,76.33 13.62,75.25 v13.62,74.53 | R46.1 C36.2 | v10.72,76.78 9.2,76.78
ENC_B
  Top 0.152: U1.34 26.24,75.98 25.74,75.48 17.3,75.48 17,75.78 U18.P$5
ENC_B_5V  (via drill 0.3)
  Top 0.2: v11.85,77.4 11.85,76.92 12.49,76.28 U18.P$3
  Bottom 0.2: v11.85,77.4 11.52,77.74 11.24,77.74 10.25,78.73 R45.1 C34.2
ENC_Z
  Top 0.152: U1.33 26.12,76.38 25.59,75.85 17.93,75.85 17,76.78 U18.P$7
ENC_Z_5V  (via drill 0.3)
  Top 0.2: U18.P$1 13,77.57 11.2,79.37 v11.2,79.83
  Bottom 0.152: 9.45,82.93 R44.1
  Bottom 0.2: R44.1 C32.2 | v11.2,79.83 11.2,81.18 9.45,82.93
ENO  (via drill 0.3)
  Top 0.152: U1.32 25.95,76.78 25.41,76.23 21.18,76.23 v20.69,76.73
  Bottom 0.152: JP1.1 19.93,81.62 20.96,80.58 20.96,77.03 20.69,76.75 v20.69,76.73
FLAG
  Top 0.152: R4.2 34.85,94.18 34.9,94.23 D1.C
  Top 0.2: X1.11 33.81,102.66 34.9,101.57 D1.C
G_HS_A  (via drill 0.35)
  Top 0.254: v22.27,47.78 22.48,47.78 22.48,48.45 U6.4 | R11.1 29.82,48.95 v29.65,48.78
  Bottom 0.2: D6.C 24,48.08
  Bottom 0.254: v22.27,47.78 22.57,48.08 24,48.08 28.95,48.08 v29.65,48.78
G_HS_B  (via drill 0.35)
  Top 0.254: v22.27,37.35 22.27,38.65 U10.4 | R9.1 29.82,38.85 v29.7,38.73
  Bottom 0.2: D7.C 24,37.75
  Bottom 0.254: 24,37.75 22.27,37.75 v22.27,37.35 | v29.7,38.73 28.73,37.75 24.23,37.75 D7.C
G_HS_C  (via drill 0.35)
  Top 0.254: U12.4 22.2,28.13 22.52,27.8 v22.52,27.23 | v29.7,28.8 29.82,28.93 R7.1
  Bottom 0.254: v22.52,27.23 22.9,27.6 D8.C 24.23,27.88 28.77,27.88 v29.7,28.8
G_HS_D  (via drill 0.35)
  Top 0.254: v22.4,17.33 22.4,18.52 U15.4 | v29.68,18.75 29.68,19.6 R5.1
  Bottom 0.2: D10.C 24,17.5
  Bottom 0.254: 24,17.5 22.45,17.5 22.4,17.45 v22.4,17.33 | D10.C 24.52,17.78 27.02,17.78 28,18.75 v29.68,18.75
G_LS_A  (via drill 0.35)
  Top 0.254: U7.4 20.57,47.13 v20.95,47.5 | R12.1 29.82,51.33 v29.75,51.25
  Bottom 0.152: R17.2 31.02,49.45 30.73,49.75
  Bottom 0.254: v20.95,47.5 20.95,48.01 21.97,49.03 28.21,49.03 29.75,50.58 | v29.75,51.25 29.75,50.58 | 29.75,50.58 29.82,50.65 30.73,49.75
G_LS_B  (via drill 0.35)
  Top 0.254: U11.4 20.8,37.13 v21,37.33 | R10.1 29.82,41.43 v29.75,41.35
  Bottom 0.152: R20.2 31.04,39.76 31.04,40.06
  Bottom 0.254: v21,37.33 22.43,38.75 26.95,38.75 29.55,41.35 v29.75,41.35 31.04,40.06
G_LS_C  (via drill 0.3, 0.35)
  Top 0.254: U13.4 20.43,27.15 v21.07,27.15 | R8.1 29.82,31.42 v29.8,31.39
  Bottom 0.152: R25.2 31.18,30.02
  Bottom 0.254: v21.07,27.15 22.68,28.75 27.16,28.75 v29.8,31.39 31.18,30.02
G_LS_D  (via drill 0.35)
  Top 0.254: v21.1,17.33 20.61,17.33 U16.4 | R6.1 29.82,21.34 v29.77,21.29
  Bottom 0.152: R28.2 31.15,19.92
  Bottom 0.254: v21.1,17.33 22.4,18.63 26.05,18.63 28.72,21.29 v29.77,21.29 31.15,19.92
GND  (via drill 0.3, 0.35)
  Top 0.152: 30.62,80.03 30.62,81.9 31.1,82.38 32.5,82.38 | 30.62,80.03 U1.77 | U1.24 29,79.98 | 29,79.98 30.57,79.98 30.62,80.03 | U1.54 33.25,74.78 31.5,76.52 | 31.42,76.78 31.59,76.61 31.5,76.52 | 31.42,76.78 30.62,77.58 30.62,78.03 | 30.62,78.03 U1.77 | U1.62 32.55,77.98 32.5,78.03 30.62,78.03 | U1.73 32.5,82.38 | U1.3 32.42,82.46 32.5,82.38 | U1.77 30,78.98 29,79.98 | U1.44 30.02,75.01 30,75.03 31.5,76.52 | U1.59 31.42,76.78
  Top 0.2: U2.4 36.92,22.05 v35.75,22.05 | U3.4 36.92,32.05 v35.75,32.05 | U4.4 36.92,42.05 v35.75,42.05 | U5.4 36.92,52.05 v35.23,52.05
  Top 0.254: v53.36,52.5 55,52.5 H4.B3,0
  other vias: 19.5,25.53 18.5,25.53 17.5,25.53 16.5,25.53 16.5,24.53 17.5,24.53 19.5,24.53 18.5,24.53 35.23,50.65 17.73,97.3 30,105.03 25,92.03 36.38,88.4 42.3,94.23 42,107.28 29.48,66.95 25.12,90.4 29.05,80.68 19,13.03 17,13.03 50.95,101.13 9.5,87.33 15.53,24.53 17.5,26.53 18.5,26.53 36.77,74 51,73.43 17.77,94.43 12.9,69.1 19.7,69.83 19.15,71.5 45.3,83.65 31.65,81.28 28.98,78.2 31.45,78.63 28.98,75.78 31.45,76.68 52,55.03 54.02,57.87 57.35,56.83 57.39,53.34 8,55.03 5.88,52.25 2.59,53.41 2.68,56.9 6.02,57.9 13.53,24.53 52,105.03 54.09,107.9 57.47,106.8 57.47,103.24 54.09,102.15 5,102.03 2.08,104.1 3.15,107.52 6.73,107.56 7.88,104.16 10.4,50.98 19,15.73 18,15.73 17,15.73 16,15.73 17.5,16.53 18.5,16.53 19.5,35.53 18.5,35.53 17.5,35.53 16.5,35.53 16.5,34.53 17.5,34.53 19.5,34.53 18.5,34.53 17.5,36.53 18.5,36.53 18.5,45.53 17.5,45.53 16.5,45.53 16.5,44.53 17.5,44.53 19.5,44.53 18.5,44.53 17.5,46.53 33.15,71.48 27.48,60 19,14.03 17,14.03 18,14.03 18,13.03 14.53,24.53 14.53,25.53 15.53,25.53 13.53,25.53 24.9,86.1 5.25,81.18 5.25,78.58 6.35,68.18 14.4,73.58 6.1,76.68 16.45,92.63 10.8,70.88 26.7,70.6 19.3,76.78 34.75,42.05 34.75,40.65 35.75,40.65 34.75,32.05 34.75,30.65 35.75,30.65 34.75,22.05 34.75,20.65 35.75,20.65 34,35.03 34,36.03 33,37.03 30,37.03 34,37.03 33,35.03 30,35.03 33,36.03 30,36.03 31,36.03 31,35.03 34.05,44.73 33.05,45.73 34.05,45.73 33.05,44.73 30.05,44.73 31.05,44.73 20.5,44.53 20.5,24.53 20.5,25.53 21.5,25.53 21.5,24.53 20.5,34.53 20.5,35.53 21.5,35.53 21.5,34.53 33.75,17.65 34.75,17.65 30.27,17.03 31.27,17.03 19.48,88.28 14.38,78.1 55.38,42 57.42,48.88 15.97,60.38 10.78,63.43 37.65,91.18 17.55,60.05 42.6,67.53 45.55,54.45 40,64.63 31.05,45.73 30.05,45.73 33.05,46.73 34.05,46.73 3.4,42.98 3.4,40.98 3.4,38.98 3.4,34.98 3.4,32.98 3.4,30.98 3.4,27.98 3.4,25.98 3.4,23.98 42.8,19.33 58,5.03 55.88,2.25 52.59,3.41 52.68,6.9 56.02,7.9 8,5.03 5.88,2.25 2.59,3.41 2.68,6.9 6.02,7.9
  pour Bottom (isolate 0.254, rank 6): 0,0.03 0,111.03 60,111.03 60,0.03
  pour Top (rank 6): 0,49 0,111.03 60,111.03 60,49
  pour Top (no thermals): 16.15,24.53 19.5,24.53 19.5,27.73 16.15,27.73
  pour Top (isolate 0.254, rank 6): 0,49.13 60,49.13 60,0.03 0,0.03
  pour Top (no thermals): 16.15,15.53 19.5,15.53 19.5,17.73 16.15,17.73
  pour Top (no thermals): 16.15,34.53 19.5,34.53 19.5,37.83 16.15,37.83
  pour Top (no thermals): 16.15,44.53 19.5,44.53 19.5,47.73 16.15,47.73
  pour Top (no thermals): 17,9.6 17,4.28 20,4.28 20,9.6
  pour Bottom (no thermals): 17,9.6 17,4.28 20,4.28 20,9.6
  pour Top (no thermals): 41,14.5 43,14.5 43,11.03 41,11.03
  pour Top (no thermals): 53.42,15.13 49.42,15.13 49.42,11.13 53.42,11.13
  pour Bottom (no thermals): 53.42,15.13 49.42,15.13 49.42,11.13 53.42,11.13
  pour Bottom (no thermals): 53.45,40.05 49.45,40.05 49.45,36.05 53.45,36.05
  pour Top (isolate 0.5, no thermals): 53.45,40.05 49.45,40.05 49.45,36.05 53.45,36.05
  cutout Bottom: 15.03,30.68 9,30.68 9,29.75 12.72,29.73 12.72,28.2 13.07,27.85 13.95,27.85 15.03,28.93
  cutout Bottom: 9.3,29.88 9.3,37.75 9.05,37.75 9.05,29.88
  pour Top (no thermals): 22,105.03 20,105.03 20,102.68 22,102.68
  pour Bottom (no thermals): 22,105.03 20,105.03 20,102.68 22,102.68
GPIO0
  Top 0.152: JP8.1 42.28,81.18 U1.70
GPIO1
  Top 0.152: JP8.2 40.14,81.58 U1.71
GPIO2
  Top 0.152: JP8.3 42.4,83.84 36.93,83.84 36.09,83 35.81,83 35.59,82.78 U1.74
GPIO3
  Top 0.152: JP8.4 37.53,84.98 35.95,83.39 35.28,83.39 35.07,83.18 U1.75
GPIO4
  Top 0.152: JP8.5 42.27,86.25 38.24,86.25 35.77,83.78 34,83.78 U1.76
GPIO5
  Top 0.152: JP8.6 38.93,87.52 35.55,84.14 U1.1
GPIO6
  Top 0.152: JP8.7 42.4,88.92 39.28,88.92 36.17,85.81 32.68,85.81 32.02,85.15 U1.4
GPIO7
  Top 0.152: JP8.8 39.87,90.06 35.99,86.19 32.55,86.19 31.62,85.25 U1.5
HALL_UX  (via drill 0.3)
  Top 0.152: U1.38 26.77,74.38 26.27,73.88 19.55,73.88 v17.3,71.63 | v11.75,72.71 11.93,72.53 U19.P$2
  Bottom 0.152: v17.3,71.63 16.15,71.63 15.27,72.51 11.95,72.51 v11.75,72.71
HALL_UX_5V  (via drill 0.3)
  Top 0.152: U19.P$6 15.35,72.03 14.55,71.23 v14.55,70.83
  Bottom 0.152: v14.55,70.83 12.2,70.83 11.25,69.88 11.25,65.93 9.35,64.03 C33.2
  Bottom 0.2: R41.1 C33.2
HALL_V
  Top 0.152: U1.37 26.62,74.78 26.09,74.25 19,74.25 16.27,71.53 U19.P$5
HALL_V_5V  (via drill 0.3)
  Top 0.152: v10.7,72.83 10.7,72.53 11.25,71.98 12.95,71.98 U19.P$3
  Bottom 0.152: C35.2 9.6,68.23
  Bottom 0.2: v10.7,72.83 10,72.13 10,68.63 9.6,68.23 | R42.1 C35.2
HALL_WY
  Top 0.152: U1.36 26.49,75.18 25.94,74.63 18.68,74.63 16.57,72.53 U19.P$7
HALL_WY_5V  (via drill 0.3)
  Top 0.152: v10.85,74.73 10.85,74.53 12.35,73.03 U19.P$1
  Bottom 0.2: v10.85,74.73 10.85,74.17 9.11,72.43 C37.2 R43.1
INPUT_GATE  (via drill 0.35)
  Top 0.5: v31.25,15.45 31.2,15.41 U22.4
  Bottom 0.5: U20.5 29.52,15.05 29.88,15.4 31.2,15.4 v31.25,15.45
MISO
  Top 0.152: X1.6 arc45 25.1,103.67 25.1,102.35 arc45 29.01,92.92 arc-45 30.02,90.47 U1.9
MOSI
  Top 0.152: U1.8 30.42,91.05 arc45 29.55,93.14 28.95,93.75 arc-45 26.52,99.62 26.52,99.92 arc90 26.18,100.25 arc-90 25.86,100.58 25.86,100.7 arc-90 26.18,101.03 26.84,101.03 arc90 27.18,101.36 27.18,101.48 arc90 26.84,101.81 26.18,101.81 arc-90 25.86,102.14 25.86,102.27 arc-90 26.18,102.6 arc90 26.52,102.93 26.52,103.43 X1.5
MOT_A  (via drill 0.35)
  Top 0.152: 21.69,49.99 v21.65,49.95
  Top 0.2: v13.6,52.23 R22.2 | U6.3 21.69,49.99
  Top 0.254: v21.65,49.95 21.1,49.95 v20.8,49.65 | U5.6 31.97,51.23 31.84,51.1 v31.69,51.1
  Bottom 0.2: U8.8 14.4,50.35 arc-100 13.6,51.15 v13.6,52.23 | 22,49.78 21.82,49.95 v21.65,49.95
  Bottom 0.254: v20.8,49.65 20.93,49.78 22,49.78 23.98,49.78 D6.A 24.15,49.95 27.18,49.95 29.3,52.08 C24.2 31.69,51.81 v31.69,51.1
  pour Top (isolate 0.305, no thermals): 22.8,53.23 22.8,49.33 21.5,49.33 20.75,48.58 15.85,48.58 15.85,53.23
  pour Top (isolate 0.305, no thermals): 12,51.4 13.3,51.4 15.82,48.88 18.7,48.88 18.7,51.13 15.88,53.95 12,53.95
MOT_A_OUT  (via drill 0.35)
  Top 0.2: v13.6,48.33 R22.1
  Bottom 0.2: v13.6,48.33 13.6,49.5 arc100 12.75,50.35 U8.1
  pour Top (isolate 0.305, no thermals): 5,46.9 5,44.03 5.42,43.6 8.3,43.6 11.28,46.58 15.18,46.58 15.18,48.28 14.1,49.35 7.45,49.35
MOT_B  (via drill 0.35)
  Top 0.152: U10.3 21.84,39.99 v21.77,39.93
  Top 0.254: v20.48,39.65 21.66,39.65 22,39.99 U10.3 | U4.6 31.97,41.23 31.84,41.1 v31.69,41.1
  Bottom 0.254: v31.69,41.1 31.69,41.81 C23.2 28.35,42.08 26,39.73 D7.A 23.93,39.65 v20.48,39.65
  pour Top (isolate 0.305, no thermals): 22.8,43.23 22.8,39.35 21.32,39.35 20.5,38.53 16.32,38.53 16.32,43.23
  pour Top (isolate 0.305, no thermals): 5,38.03 5,36.6 5.58,36.03 10.1,36.03 12.7,38.63 20,38.63 20,43.03 12.25,43.03 8.95,39.73 6.7,39.73
MOT_C  (via drill 0.35)
  Top 0.2: v13.6,32.55 R21.2
  Top 0.254: v20.1,29.65 20.44,29.99 v21.82,29.99 U12.3 | U3.6 31.97,31.23 31.84,31.1 v31.69,31.1
  Bottom 0.2: U9.8 14.38,30.55 arc-100 13.6,31.33 v13.6,32.55 | 22,29.8 21.82,29.98 v21.82,29.99
  Bottom 0.254: v20.1,29.65 20.25,29.8 22,29.8 D8.A 26.68,29.8 28.95,32.08 C22.2 31.69,31.81 v31.69,31.1
  pour Top (isolate 0.305, no thermals): 22.77,33.4 22.77,29.33 21.3,29.33 20.5,28.53 16.3,28.53 16.3,33.4
  pour Top (isolate 0.305, no thermals): 11.93,34.03 15.2,34.03 15.88,33.35 16.32,33.35 16.52,33.15 17.45,33.15 17.45,28.65 16,28.65 13.05,31.6 11.93,31.6
MOT_C_OUT  (via drill 0.35)
  Top 0.2: v13.6,28.6 R21.1
  Bottom 0.2: U9.1 12.7,30.55 arc-100 13.6,29.65 v13.6,28.6
  pour Top (isolate 0.305, no thermals): 15.2,26.8 6.58,26.8 5,28.38 5,30.03 5.78,30.8 12.82,30.8 14.93,28.7 15.1,28.7 15.2,28.6
MOT_D  (via drill 0.35)
  Top 0.254: v20.07,19.2 20.86,19.99 v21.77,19.99 U15.3 | U2.6 31.97,21.23 31.84,21.1 v31.69,21.1
  Bottom 0.2: 22,19.45 21.77,19.68 v21.77,19.99
  Bottom 0.254: v20.07,19.2 20.32,19.45 22,19.45 D10.A 25.75,19.45 28.5,22.2 31.3,22.2 C21.2 31.69,21.81 v31.69,21.1
  pour Top (isolate 0.305, no thermals): 22.8,23.23 22.8,19.4 21.38,19.4 20.6,18.63 16.5,18.63 16.5,23.23
  pour Top (isolate 0.305, no thermals): 21,19.03 6,19.03 5,20.03 5,22.53 5.75,23.28 21,23.28
N$1
  Top 0.2: R37.1 7.9,68.23 3.6,63.93 3.06,63.93 JP12.4
  Bottom 0.2: R41.2 5.29,63.99 JP12.4
N$3
  Top 0.2: R39.1 7.9,71.53 5.4,69.03 5.4,67.73 4.2,66.53 JP12.3
  Bottom 0.2: R42.2 3.4,66.13 JP12.3
N$4  (via drill 0.3)
  Top 0.152: v28.5,87.33 28.82,87.01 U1.12
  Top 0.2: D1.A 34.9,87.68 v34.98,87.6
  Bottom 0.2: v34.98,87.6 34.04,86.66 29.16,86.66 v28.5,87.33
N$5  (via drill 0.35)
  Top 0.2: v44.15,54.7 44.15,55.55 U24.3 42.58,55.85 R49.1
  Bottom 0.2: R50.2 44.15,54.95 v44.15,54.7
N$6
  Bottom 0.254: R23.2 21.25,62.2 15.65,56.6 U8.5
N$7  (via drill 0.3)
  Top 0.2: JP11.4 6.44,77.49 R38.1 6.9,76.03 v6.3,75.43
  Bottom 0.2: R46.2 6.45,75.43 v6.3,75.43
N$8
  Top 0.2: LED1.A 19.15,99.23 R34.1
N$9  (via drill 0.3)
  Top 0.2: R36.1 7.4,78.13 v6.6,78.93 5.5,80.03 JP11.3
  Bottom 0.2: R45.2 6.8,78.73 v6.6,78.93
N$10
  Bottom 0.254: R24.2 23.5,62.75 17.68,56.93 17.68,49.48 15.25,47.05 15.25,32.9 U9.5
N$11  (via drill 0.3)
  Top 0.2: R35.1 7.9,81.33 6.6,82.63 6.5,82.63 | 6.5,82.63 3.06,82.63 JP11.2 | v6.5,82.83 6.5,82.63
  Bottom 0.2: R44.2 6.6,82.93 v6.5,82.83
N$12
  Top 0.5: D14.A 39.76,61.53
  Top 0.75: U24.1 44.45,58.8 43.17,60.08 43.17,60.8 L2.2
  Top 1: L2.2 42.45,61.53 39.76,61.53
N$13
  Top 0.254: U5.5 31.52,52.03 R12.2
N$15  (via drill 0.3)
  Top 0.2: R40.1 6.8,72.83 6.8,71.93 6.25,71.38 | 6.25,71.38 3.94,69.07 JP12.2 | v6.5,71.13 6.25,71.38
  Bottom 0.2: R43.2 6.55,71.13 v6.5,71.13
N$16  (via drill 0.35)
  Top 0.5: 49.2,44.9 49.23,44.92 U23.8 50.13,44.32 v50.8,43.65
  Top 0.8: 45.95,45.65 L1.1 | 46.7,44.9 46.63,44.97 45.95,45.65 | 45.95,45.65 45.67,45.93
  Top 1: 49.2,44.9 46.7,44.9 | D12.C 44.84,45.1 45.67,45.93
  Bottom 0.2: C42.2 51.6,42.85 v50.8,43.65
N$17
  Top 0.2: X1.16 38.89,106.14 40.35,104.68 40.35,102.38 39.05,101.08 R31.2
N$18  (via drill 0.35)
  Top 0.254: v32.65,48.78 32.65,49.57 32.71,49.63 U5.8
  Bottom 0.25: v32.65,48.78 33.15,48.78 33.7,49.33 D5.C
  Bottom 0.254: C24.1 33.52,51.88 33.52,49.66 D5.C
N$19  (via drill 0.35)
  Top 0.2: v56.38,44.55 56.38,44.7 56.16,44.92 U23.1
  Bottom 0.2: v56.38,44.55 54.67,42.85 C42.1
N$20
  Top 0.5: SJ4.1 22.38,99.69 22.38,104.5 23.65,105.78 X1.4
N$21  (via drill 0.35)
  Top 0.2: v49.05,48.85 49.15,48.75 50.11,48.75 U23.5
  Bottom 0.2: R48.1 53.55,49.3 51.73,49.3 51.75,49.28 R47.1 51.55,48.73 49.17,48.73 v49.05,48.85
N$22
  Top 0.2: JP3.2 JP3.4 JP3.6
  Bottom 0.2: R32.1 R33.2 12.67,99.48 JP3.2
N$23
  Top 1: X1.2 20.41,107 13.65,107 JP5.1
N$24
  Bottom 0.5: U20.1 25.55,14.1 25.55,12.38 C39.1
N$25  (via drill 0.35)
  Top 0.2: v56.42,46.2 56.42,46.12 56.4,46.09 55.67,46.09 U23.2
  Bottom 0.2: C41.2 54.88,46.1 56.33,46.1 v56.42,46.2
N$27
  Top 0.254: U5.7 32.2,50.43 R11.2
N$28  (via drill 0.35)
  Top 0.254: U4.8 32.65,39.22 v32.65,38.78
  Bottom 0.254: v32.65,38.78 33.33,39.45 33.45,39.45
  Bottom 0.3: C23.1 33.35,42.05 33.35,39.55 33.45,39.45 33.58,39.33 D4.C
N$29
  Top 0.254: U4.5 31.52,42.03 R10.2
N$30
  Top 0.254: U4.7 32.2,40.43 R9.2
N$31  (via drill 0.35)
  Top 0.254: v32.65,18.78 32.65,19.57 32.71,19.63 U2.8
  Bottom 0.254: v32.65,18.78 33.2,19.33 D2.C
  Bottom 0.3: C21.1 33.55,21.85 33.55,19.33 D2.C
N$32
  Top 0.254: U2.5 31.52,22.03 R6.2
N$33
  Top 0.254: U2.7 32.2,20.43 R5.2
N$34  (via drill 0.35)
  Top 0.254: v32.65,28.78 32.65,29.57 32.71,29.63 U3.8
  Bottom 0.254: v32.65,28.78 33.2,29.33 D3.C
  Bottom 0.3: C22.1 33.48,31.93 33.48,29.33 D3.C
N$35
  Top 0.254: U3.5 31.52,32.03 R8.2
N$36
  Top 0.254: U3.7 32.2,30.43 R7.2
PWM_I
  Top 0.152: JP10.1 56.31,76.38 U1.58
REF_H
  Top 0.152: JP9.3 56.23,84.29 56.23,86.27 55.31,87.19 54.07,87.19 47.26,80.38 U1.68
REF_L
  Top 0.152: JP9.1 55.8,82.18 55.8,86.19 55.16,86.83 54.26,86.83 47.4,79.98 U1.67
REF_R
  Top 0.152: JP9.5 55.52,87.54 53.81,87.54 47.04,80.78 U1.69
RES_FET  (via drill 0.35)
  Top 0.254: v39,15.03 37.83,13.85 U17.5
  Bottom 0.254: D11.A 41,15.25
  Bottom 0.305: 41,15.25 39.23,15.25 v39,15.03
  Bottom 1: D15.C 41.43,10.44 X2.4
  pour Top (isolate 0.305, no thermals): 42.5,9.03 42.5,5.53 42,5.03 41.02,5.03 35.75,10.3 35.75,15.6 40,15.6 40,11.03 42,9.03
RESET  (via drill 0.3)
  Top 0.152: U1.50 32.4,73.78 32.4,69.19 v32.66,68.93 | X1.3 23.65,89.15 v23.6,89.15
  Top 0.2: v21.68,72.28 21.7,72.28 21.7,69.03 v21.6,68.93
  Bottom 0.152: v23.6,89.15 23.6,89.08
  Bottom 0.2: v32.66,68.93 28,68.93 | 28,68.93 24.86,68.93 24.85,68.93 v21.6,68.93 | 23.6,89.08 23.5,88.98 23.5,85.45 21.88,83.83 21.88,72.73 21.68,72.53 v21.68,72.28 | R3.1 28.02,68.95 28,68.93
SCK
  Top 0.152: U1.7 30.82,91.02 arc45 29.7,93.73 29.36,94.07 arc-45 27.57,98.37 27.57,105.07 arc-45 27.79,105.58 28.5,106.3 X1.8
SENSE_A  (via drill 0.3)
  Top 0.152: U1.16 26.8,83.18 25.2,84.78 v24.6,84.78
  Top 0.2: v23,71.85 23,67.05 v22.75,66.8
  Bottom 0.2: v24.6,84.78 24.02,84.78 23.3,84.05 23.3,72.15 v23,71.85 | C30.2 R23.1 21.25,65.78 22.27,66.8 v22.75,66.8
SENSE_C  (via drill 0.3)
  Top 0.152: U1.18 26.04,82.38 25.09,83.33 v24.19,83.33 v24.18,83.32
  Top 0.2: v23.65,66.18 23.68,66.2 23.68,71.1 v23.75,71.18
  Bottom 0.152: v24.18,83.32 24.21,83.29
  Bottom 0.2: 24.21,83.29 23.71,82.79 23.71,71.22 v23.75,71.18 | C31.2 R24.1 23.65,64.98 v23.65,66.18
STEP
  Top 0.152: JP10.2 55.55,75.98 U1.57
UART_RX  (via drill 0.3)
  Top 0.152: U1.10 29.62,90.15 arc45 28.84,92.04 26.65,94.23 v25.15,94.23
  Top 0.2: JP6.1 56.38,97.95 v43.12,97.95
  Bottom 0.2: v25.15,94.23 28.88,97.95 v43.12,97.95
UART_TX  (via drill 0.3)
  Top 0.152: U1.11 29.22,89.91 arc45 28.55,91.52 26.85,93.23 v25.15,93.23
  Top 0.2: JP6.2 54.77,97.03 v42,97.03
  Bottom 0.2: v42,97.03 41.77,97.26 29.18,97.26 v25.15,93.23
V+  (via drill 0.35)
  Top 0.4: U23.7 49.06,46.19 v49.02,46.23
  Top 0.5: v27.88,16.73 27.8,16.65 27.8,14.88 U22.5
  Top 0.8: C12.+ 53.98,32.94 53.98,39.15 52.12,41 52.12,44.82 50.75,46.19 U23.7
  Bottom 0.2: R13.2 24.15,52.85 v24.23,52.78 | R47.2 51.2,46.48 49.27,46.48 v49.02,46.23 48.8,46.23 47.08,47.95 47.08,67.83 R15.2
  Bottom 0.305: v41.17,24 41.17,18.99 D11.C
  Bottom 0.5: v27.88,16.73 U20.4 | v49.02,46.23 49.02,45.98 C43.2
  other vias: 24.9,22.18 24.9,21.38 24.2,21.08 24.2,22.48 24.88,32.45 24.88,31.65 24.18,31.35 24.18,32.75 24.9,42.28 24.9,41.48 24.2,41.18 24.2,42.58 24.93,52.48 24.93,51.68 24.23,51.38
  pour Bottom (isolate 0.305, no thermals): 23.73,51.18 23.73,52.98 25.23,52.98 25.23,51.18
  pour Bottom (isolate 0.305, no thermals): 23.7,20.73 23.7,22.8 25.2,22.8 25.2,20.73
  pour Bottom (isolate 0.305, no thermals): 23.68,31.15 23.68,32.95 25.18,32.95 25.18,31.15
  pour Bottom (isolate 0.305, no thermals): 23.7,40.98 23.7,42.78 25.2,42.78 25.2,40.98
  pour Top (isolate 0.5, no thermals): 23.27,53.03 29,53.03 29,7.03 27,5.03 25.48,5.03 23.27,7.23
  pour Top (no thermals): 53.42,20.55 53.42,30.73 52.17,31.98 50.67,31.98 49.42,30.73 49.42,28.13 28,28.13 28,23.48 49.42,23.48 49.42,20.6 50.67,19.35 52.23,19.35
V_EXT  (via drill 0.3)
  Top 0.2: X1.13 36.35,103.25 37.1,102.5 37.1,92.95 37.92,92.13 45.9,92.13 v46.17,91.85
  Bottom 0.2: R19.2 45.5,73.08 46.4,73.98 46.4,91.63 v46.17,91.85
  Bottom 0.3: R18.1 R19.2
V_GD  (via drill 0.35)
  Top 0.2: R49.2 41.75,56.93
  Top 0.254: U5.1 36.97,49.65 v38.17,49.65 38.08,49.65 37.98,49.55 C10.2 | U4.1 v38.15,39.63 38.17,39.65 C9.2 | U3.1 v38.15,29.63 38.2,29.58 C8.2 | U2.1 v38.15,19.63 38.15,20 39.52,21.38 C7.2
  Top 0.3: U14.2 40.67,21.1 C7.2
  Top 0.5: 37,58.3 C45.1 37.27,58.18 | 41.75,56.93 40.44,58.24 D14.C 39.69,58.18
  Top 1: 39.69,58.18 37.27,58.18 | JP4.1 34.65,58.3 37,58.3
  Bottom 0.2: D5.A 36.87,49.06 36.87,49.03
  Bottom 0.254: v38.17,49.65 37.85,49.33 D5.A | v38.15,39.63 37.85,39.33 D4.A | v38.15,29.63 37.85,29.33 D3.A | v38.15,19.63 37.85,19.33 D2.A
  Bottom 1: D2.A 37.17,19.33 37.17,29.33 D3.A 37.14,29.63 D4.A 36.87,39.6 36.87,49.03 36.87,57.16 33.95,60.08 JP4.1
V_INT  (via drill 0.3)
  Top 0.2: X1.14 37.6,105.05 37.6,93.03 37.98,92.65 46.84,92.65 v46.93,92.55
  Bottom 0.2: R16.2 48,73.05 47.05,74 47.05,92.43 v46.93,92.55
  Bottom 0.3: R16.2 R15.1
V_INT_TMC  (via drill 0.3)
  Top 0.152: v24.4,72.68 24.4,72.5 24.88,72.03 24.88,60.9 v24.5,60.53 | U1.20 25.2,81.58 v24.93,81.85
  Bottom 0.152: v24.5,60.53 23.88,60.53 22.75,59.4 C25.1 | v24.93,81.85 24.27,81.85 24.27,72.75 24.35,72.68 v24.4,72.68
  Bottom 0.2: C25.1 R14.2 22.5,56.5 22.5,54.78 R13.1
V_MOT_IN  (via drill 0.35)
  Bottom 0.2: X2.3 33.81,10.41 36.58,13.18 41.77,13.18 46.35,17.75 46.35,67.88 R18.2 | U20.3 26.02,16 26.52,15.5 26.52,14.36 26.78,14.1 U20.6
  Bottom 0.5: v30.43,13.85 30.18,14.1 U20.6 27.53,14.1 27.53,12.46 C39.2
  other vias: 31.43,13.85 30.43,12.85 32.42,12.85 31.43,12.85 30.43,11.85
  pour Top (isolate 0.4, no thermals): 29.7,14.5 29.7,6.23 30.9,5.03 34.38,5.03 34.8,5.45 34.8,8.6 34,9.4 34,12.1 31.6,14.5
  pour Bottom (isolate 0.4, no thermals): 29.7,14.5 29.7,6.23 30.9,5.03 34.38,5.03 34.8,5.45 34.8,11.3 31.6,14.5
V_SENSE/2  (via drill 0.3, 0.35)
  Top 0.152: U1.17 26.44,82.78 25.19,84.03 23.12,84.03 C2.2 22.62,84.38 v22.62,83.5 23.52,82.6 25.09,82.6 25.72,81.98 U1.19
  Top 0.2: v22.63,72.72 22.33,72.42 22.33,68.15 22.02,67.85 22.02,66.28 v22.41,65.89 | v16.68,55.55 16.52,55.7 12.09,55.7 v11.96,55.83
  Bottom 0.15: 13.4,33.5 13.4,34.98
  Bottom 0.152: U9.3 12.32,31.85 12.67,32.2 12.67,32.85 13.32,33.5 13.4,33.5 13.85,33.5 14.31,33.04 14.31,32.07 15.02,31.36 15.49,31.36 U9.7 | R1.1 12.07,56.68 | 13.48,55.27 13.48,53.43 | 13.48,53.43 13.48,53.4 13.74,53.4 14.34,52.8 14.34,51.43 14.62,51.16 15.49,51.16 U8.7 | 13.48,53.43 12.5,52.44 12.5,52.09 12.06,51.65 U8.3 | C1.2 14.12,43.8
  Bottom 0.2: U8.7 16.38,51 16.57,50.8 16.57,49.87 14.12,47.42 14.12,43.8 14.12,35.7 13.4,34.98 | v22.62,83.5 22.73,83.4 22.73,72.81 v22.63,72.72 | v22.41,65.89 22.39,65.86 22.39,62.39 16.68,56.68 v16.68,55.55 | 13.48,55.27 12.44,56.31 | 12.44,56.31 12.07,56.68 | v11.96,55.83 12.44,56.31
  Bottom 0.3: R2.2 R1.1
VCORE  (via drill 0.3)
  Top 0.152: v30.15,71.71 30.15,71.78 30.42,72.05 U1.45 | U1.15 27.04,83.58 26.87,83.75 v26.87,84.93 | v35.62,78.13 35.38,78.38 U1.63
  Bottom 0.152: C5.2 26.87,84.41 v26.87,84.93 | v35.62,78.13 35.62,78.55 C6.2
  Bottom 0.2: v30.15,71.71 30.15,71.78 C3.2 30.93,72.8 30.3,73.43 30.3,75.88 29.4,76.78 27.43,76.78 26.77,77.43 26.77,83.33 27.07,83.63 C5.2 30.77,80.5 34.08,80.5 35.02,79.55 C6.2

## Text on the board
tPlace: 5V | E-Stop | EN | GND | 3V3 | P | N | Jumper / (Single ended) | V | AENC | RX | U | TX | W | GND | 5V | 7 | 6 | UART (3V3) | 3V3 | 2V5 / N Offset | GND | 4 | 5 | 5V | R | AGPI_A | GPIO | 3 | 2 | Z | Z | 0 | B | H | ENC | ENO | 1 | L | B | ENC2 (3V3) | A | TMC4671 | A | PWM | GND | STP | 5V | DIR | WY | V | HALL | UX | GND | 5V | 10V | A | MOTOR | B | C | D | 3 phase / ABC = UVW | MOTOR / A|B|C|D | GND | PB+ | VM | PB- | Power | SUPPLY / 1:GND / 2:PB+ / 3:VM + / 4:PB-
bPlace: 5V | E-Stop | 16 | 2 | 1 | GND | 5V | RST | 3V3 | MOSI | MISO | CS1 | SCK | CS2 | CS3 | FLAG | BRK | V_EXT | V_INT | NC | ENABLE | EN | GND | P | N | V | RX | UART | U | TX | Cos | 1 | 2 | 3 | AENC | GND | W | Sin | N/CM | 2V5 | 3V3 | 5V | N Offset | SPI ADDR | 5V | GND | ENC2 (3V3) | Z | R | 5V | B | H | Z | A | L | B | ENC | PWM | A | STP | GND | DIR | 5V | WY | V | HALL | UX | GND | V_GD / (10V) | 5V | STEPPER: AB(A) CD(B) | 3 PHASE: ABC(UVW) | DC: AB | Open FFBoard - TMC4671 Motor driver | TMP | A | B | MOTOR | C | D | V1.2.1 - YR 2021 | Supply: / PSU (protected): VM (+) and GND (-) / ALWAYS use braking resistor between PB+ and PB / / Battery: PB+ (+) and GND (-) No resistor | R | VM | GND | PB+ | PB- | - | + | Power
